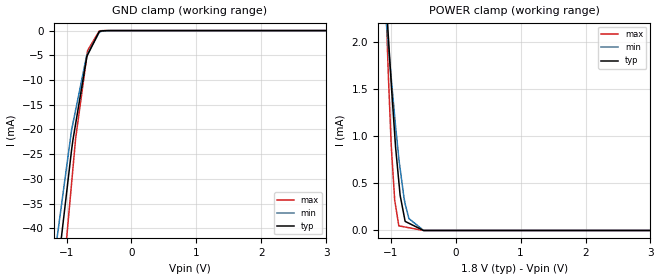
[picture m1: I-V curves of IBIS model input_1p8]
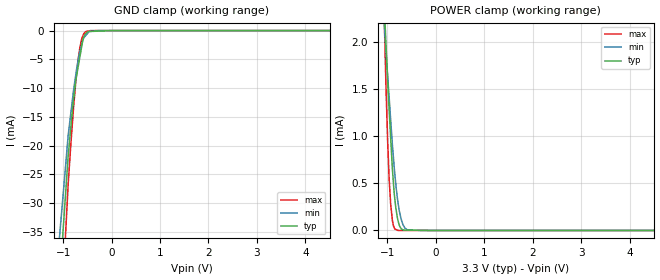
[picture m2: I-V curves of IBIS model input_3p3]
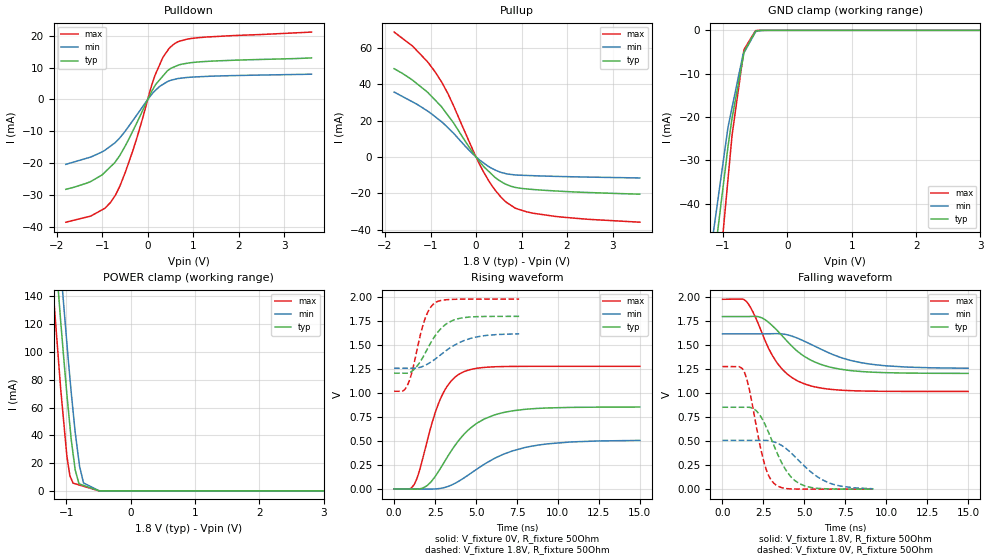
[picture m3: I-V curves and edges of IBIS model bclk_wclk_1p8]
|Texas Instruments Incorporated
| Low-Power Stereo DAC with 4 Outputs, HP/Speaker Amplifier and 3D Effects
| Marketing part#   Digital Voltage Range   Package-type   #pins
| TLV320DAC32IRHBR   1.1V - 3.6V   QFN   32
| TLV320DAC32IRHBRG4  1.1V - 3.6V   QFN   32
| TLV320DAC32IRHBT   1.1V - 3.6V   QFN   32
| TLV320DAC32IRHBTG4  1.1V - 3.6V   QFN   32
[IBIS Ver]   3.2
[File name]   tlv320dac32.ibs
|SIMDE Ver   V3.0 - 201101 - RHL4 - Build 457
[File Rev]   1.0
[Date]   9/15/2011
[Source]
| Texas Instruments Incorporated.
| Analog-eLab Design Center, HPA
| 12500 TI Blvd
| Dallas, TX -75243
| e-mail: elab_scm_ibis@list.ti.com
[Notes]   Revision History:
| Rev 1.0: 9/15/2011
| - Initial version of the model
| - Model generated from simulations in TISPICE
| - Model matched to SPICE simulation
| - C_comp although listed in numerical order of value are
|   obtained from varying PVT conditions. For PVT conditions for
|   each specific value refer the buffer description under
|   respective [Model]. IBIS model user is responsible for using
|   appropriate C_comp to simulate for Signal Integrity.
| - Model names with a trailing _1p8 contains the model for
|   1.8V [1.62V and 1.98V].Model names with a trailing _3p3
|   contains the model for 3.3V [3.0V and 3.6V].
[Disclaimer]
| This model is designed as an aid for customers of Texas Instruments.
| TI and its licensors and suppliers make no warranties, either expressed
| or implied, with respect to this  model, including the warranties of
| merchantability or fitness for a particular purpose. The model is
| provided solely on an "as is" basis. The entire risk as to its quality
| and performance is with the customer.
[Copyright]
 (C) Copyright 2011 Texas Instruments Incorporated.All rights reserved.
|   TLV320DAC32RHB
[Component]   TLV320DAC32RHB
[Manufacturer]   TI
[Package]   |32 QFN  -  RHB package
|   typ   min   max
R_pkg   0.09398   0.03334   0.13311
L_pkg   1.47574nH   0.53442nH   2.12719nH
C_pkg   0.15630pF   0.08976pF   0.19319pF
[Pin]  signal_name   model_name   R_pin   L_pin   C_pin
1   MCLK   INPUT   0.12336   1.96644nH  0.15900pF
2   BCLK   BCLK_WCLK   0.10740   1.68468nH  0.14850pF
3   WCLK   BCLK_WCLK   0.10191   1.58900nH  0.14672pF
4   DIN   INPUT   0.10100   1.57299nH  0.14533pF
5   LDO_SELECT   INPUT   0.10460   1.63539nH  0.15162pF
6   IOVSS   GND   0.11459   1.80939nH  0.15817pF
7   IOVDD   POWER   0.10859   1.70548nH  0.15212pF
8   SCL   SCL   0.12335   1.96583nH  0.16003pF
9   SDA   SDA   0.11930   1.89434nH  0.14528pF
10   LINEL   TERM   0.00029   0.05488nH  0.04405pF
11   LINEL   TERM   0.05460   0.78769nH  0.08976pF
12   LINEL   TERM   0.03334   0.53442nH  0.16822pF
13   LINER   TERM   0.03421   0.55249nH  0.17502pF
14   LINER   TERM   0.00029   0.05440nH  0.04408pF
15   MICBIAS   TERM   0.03710   0.57816nH  0.18724pF
16   MICBIAS   TERM   0.00029   0.05754nH  0.03663pF
17   DRVSS   GND   0.13014   2.07654nH  0.15925pF
18   DRVDD   POWER   0.05310   1.27721nH  0.19416pF
19   HPLOUT   TERM   0.10102   1.56409nH  0.15141pF
20   HPLCOM   TERM   0.10193   1.57999nH  0.15153pF
21   DRVSS   GND   0.05419   1.31855nH  0.20715pF
22   HPRCOM   TERM   0.11859   1.87140nH  0.17545pF
23   HPROUT   TERM   0.13311   2.12719nH  0.19319pF
24   DRVDD   POWER   0.07565   2.22477nH  0.22198pF
25   AVDD_DAC   POWER   0.12099   1.91764nH  0.14964pF
26   AVSS_DAC   GND   0.03485   0.58219nH  0.16642pF
27   AVSS_DAC   GND   0.00029   0.05439nH  0.04408pF
28   AVSS_DAC   GND   0.05222   0.75975nH  0.08772pF
29   AVSS_DAC   GND   0.05222   0.75975nH  0.08756pF
30   AVSS_DAC   GND   0.05686   0.82975nH  0.09264pF
31   _RESET   INPUT   0.10879   1.70768nH  0.15255pF
32   DVDD   POWER   0.06209   1.75808nH  0.19293pF
33   THERMAL_PAD   NC   0.00003   0.01397nH  0.12486pF
[Pin Mapping]  pulldown_ref pullup_ref gnd_clamp_ref power_clamp_ref
1   GNDBUS1   PWRBUS1
2   GNDBUS1   PWRBUS1
3   GNDBUS1   PWRBUS1
4   GNDBUS1   PWRBUS1
5   GNDBUS1   PWRBUS1
6   GNDBUS1   NC
7   NC   PWRBUS1
8   GNDBUS1   PWRBUS1
9   GNDBUS1   PWRBUS1
10   GNDBUS2   PWRBUS2
11   GNDBUS2   PWRBUS2
12   GNDBUS2   PWRBUS2
13   GNDBUS2   PWRBUS2
14   GNDBUS2   PWRBUS2
15   GNDBUS2   PWRBUS2
16   GNDBUS2   PWRBUS2
17   GNDBUS2   NC
18   NC   PWRBUS2
19   GNDBUS2   PWRBUS2
20   GNDBUS2   PWRBUS2
21   GNDBUS2   NC
22   GNDBUS2   PWRBUS2
23   GNDBUS2   PWRBUS2
24   NC   PWRBUS2
25   NC   PWRBUS3
26   GNDBUS3   NC
27   GNDBUS3   NC
28   GNDBUS3   NC
29   GNDBUS3   NC
30   GNDBUS3   NC
31   GNDBUS1   PWRBUS1
32   NC   PWRBUS4
33   NC   NC
|   Model Selectors
[Model Selector] INPUT
input_1p8   1.8V digital input
input_3p3   3.3V digital input
[Model Selector] BCLK_WCLK
bclk_wclk_1p8   1.8V digital I/O
bclk_wclk_3p3   3.3V digital I/O
[Model Selector] SCL
scl_1p8   1.8V digital input
scl_3p3   3.3V digital input
[Model Selector] SDA
sda_1p8  1.8V digital I/O_open_drain
sda_3p3  3.3V digital I/O_open_drain
[Model Selector] TERM
term_1-8V  1.8V nominal termination
term_3-3V  3.3V nominal termination
[Model] term_1-8V
Model_type Terminator
C_comp   1.0e-20F  1.0e-20F  1.0e-20F
|   typ   min   max
[Voltage Range]   1.8V   1.62V   1.98V
[POWER Clamp Reference]   1.8V   1.62V   1.98V
[GND Clamp Reference]   0V   0V   0V
|Ambient Temperature   25   85   -40
|Junction Temperature
[Temperature Range]   45   105   -40
[Model] term_3-3V
Model_type Terminator
C_comp   1.0e-20F  1.0e-20F  1.0e-20F
|   typ   min   max
[Voltage Range]   3.3V   3.0V   3.6V
[POWER Clamp Reference]   3.3V   3.0V   3.6V
[GND Clamp Reference]   0V   0V   0V
|Ambient Temperature   25   85   -40
|Junction Temperature
[Temperature Range]   45   105   -40
| Models and submodels in the file (10): input_1p8 (Input), input_3p3 (Input), bclk_wclk_1p8 (I/O), bclk_wclk_3p3 (I/O), scl_1p8 (Input), scl_3p3 (Input), sda_1p8 (I/O_open_drain), sda_3p3 (I/O_open_drain), term_1-8V (Terminator), term_3-3V (Terminator)
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|   input_1p8 Model
[Model]   input_1p8
Model_type   Input
Vinl = 0.54
Vinh = 1.26
|   typ   min   max
|   (nom PVT)   (fast PVT)   (slow PVT)
|C_comp from frequency sweep method (F=50MHz)
|Average
|C_comp   1.487e-12   1.450e-12   1.504e-12
|C_comp from LC tank measurement(L=1nH)
|Average
|Resonant Frequency(Hz)   4.930e+09   4.940e+09   4.930e+09
C_comp   1.043e-12   1.039e-12   1.043e-12
[Model spec]
|subparameter   typ   min   max
Vinl   0.54   0.486   0.594
Vinh   1.26   1.134   1.386
| Where nom  PVT is Nominal Process, 1.8V, 45C
|   Fast PVT is Strong Process,  1.98V, -40C
|   Slow PVT is Weak Process,   1.62V, 105C
[Voltage Range]   1.8   1.62   1.98
|Ambient Temperature   25   85   -40
|Junction Temperature
[Temperature Range]   45   105   -40
[Power Clamp Reference]   1.8   1.62   1.98
[GND Clamp Reference]   0   0   0
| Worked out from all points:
|   GND clamp passes 1 mA (typ) near -0.53 V on its own axis
|   POWER clamp passes 1 mA (typ) near -0.94 V on its own axis
[GND Clamp]
|   Voltage   I(typ)   I(min)   I(max)
-1.8V     -206.9mA   -110.5mA   -320.4mA
-1.152V   -50.18mA   -42.62mA   -64.48mA
-923.4mV  -24.31mA   -20.25mA   -31.11mA
-901.8mV  -22.19mA   -18.82mA   -27.97mA
-859.3mV  -18.84mA   -16.06mA   -21.82mA
-690.1mV  -5.53mA    -5.064mA   -5.476mA
-685.8mV  -5.19mA    -4.959mA   -5.059mA
-675.2mV  -4.913mA   -4.7mA     -4.033mA
-495mV    -199uA     -315.9uA   -54.51uA
-426.1mV  -36.83uA   -68.97uA   -5.36uA
-307.8mV  -1.051uA   -3.83uA    -71.36nA
3.6V      0A         0A         0A
[POWER Clamp]
|   Voltage   I(typ)   I(min)   I(max)
-1.8V     11.87mA    8.619mA    19.35mA
-1.085V   2.649mA    2.361mA    2.616mA
-1.039V   2.086mA    1.979mA    1.704mA
-990mV    1.542mA    1.604mA    881.4uA
-938.5mV  1.023mA    1.21mA     323.2uA
-923.4mV  874.4uA    1.094mA    257.8uA
-875.2mV  522uA      770.1uA    49.36uA
-855mV    374.8uA    656.9uA    46.74uA
-777.6mV  96.52uA    281.9uA    36.69uA
-719.3mV  76.6uA     126.4uA    29.12uA
-494.1mV  11.66nA    505.2nA    0A
3.6V      0A         0A         0A
|   input_3p3 Model
[Model]   input_3p3
Model_type   Input
Vinl = 0.99
Vinh = 2.31
|   typ   min   max
|   (nom PVT)   (fast PVT)   (slow PVT)
|C_comp from frequency sweep method (F=50MHz)
|Average
|C_comp   1.401e-12   1.371e-12   1.413e-12
|C_comp from LC tank measurement(L=1nH)
|Average
|Resonant Frequency(Hz)   5.100e+09   5.110e+09   5.090e+09
C_comp   9.748e-13   9.710e-13   9.787e-13
[model spec]
|subparameter   typ   min   max
Vinl   0.99   0.90   1.08
Vinh   2.31   2.10   2.52
| Where nom  PVT is Nominal Process, 3.3V, 45C
|   Fast PVT is Strong Process,  3.6V, -40C
|   Slow PVT is Weak Process,   3V, 105C
[Voltage Range]   3.3   3   3.6
|Ambient Temperature   25   85   -40
|Junction Temperature
[Temperature Range]   45   105   -40
[Power Clamp Reference]   3.3   3   3.6
[GND Clamp Reference]   0   0   0
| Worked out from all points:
|   GND clamp passes 1 mA (typ) near -0.57 V on its own axis
|   POWER clamp passes 1 mA (typ) near -0.93 V on its own axis
[GND Clamp]
|   Voltage   I(typ)   I(min)   I(max)
-3.3V     -1.459A    -1.317A    -1.646A
-1.49V    -95.13mA   -76.77mA   -122mA
-897.6mV  -21.78mA   -18.26mA   -26.74mA
-792mV    -12.42mA   -10.77mA   -14.02mA
-745.8mV  -8.948mA   -8.013mA   -9.431mA
-702mV    -6.825mA   -5.63mA    -5.815mA
-622.8mV  -2.986mA   -2.616mA   -1.616mA
-590.7mV  -1.43mA    -1.587mA   -839.1uA
-532.8mV  -508.5uA   -839.9uA   -172.5uA
-465mV    -161.8uA   -161.4uA   -53.2uA
-285mV    -98.74uA   -2.083uA   -3.877uA
6.6V      0A         0A         0A
[POWER Clamp]
|   Voltage   I(typ)   I(min)   I(max)
-3.3V     32.08mA    22.4mA     56.05mA
-1.089V   2.679mA    2.39mA     2.744mA
-1.03V    1.983mA    1.906mA    1.532mA
-993.6mV  1.586mA    1.634mA    934uA
-964.8mV  1.288mA    1.419mA    561.5uA
-932.4mV  983.8uA    1.176mA    280.4uA
-896.4mV  648.9uA    907.5uA    104uA
-864.6mV  429.3uA    705.3uA    36.05uA
-792mV    130.4uA    335uA      1.308uA
-681mV    8.006uA    64.67uA    29.85nA
-585mV    3.401uA    6.441uA    18.01nA
6.6V      0A         0A         0A
|   bclk_wclk_1p8 Model
[Model]   bclk_wclk_1p8
Model_type   I/O
Polarity   Non-Inverting
Enable   Active-Low
Vinl = 0.54
Vinh = 1.26
Vmeas = 0.9
Vref = 0.9
Cref = 10pF
Rref = 50
|   typ   min   max
|   (nom PVT)   (fast PVT)   (slow PVT)
|C_comp from frequency sweep method (F=14MHz)
|Average
|C_comp   3.261e-12   3.029e-12   3.353e-12
|ON state : BUFFER OUTPUT TURNED HIGH
|C_comp   4.573e-12   4.126e-12   4.742e-12
|OFF state: BUFFER IN HIGH IMPEDANCE
|C_comp   1.949e-12   1.931e-12   1.963e-12
|C_comp from LC tank measurement(L=1nH)
|Average
|Resonant Frequency(Hz)   4.330e+09   4.360e+09   4.290e+09
|C_comp   1.354e-12   1.336e-12   1.381e-12
|ON state : BUFFER OUTPUT TURNED HIGH
|Resonant Frequency(Hz)   4.230e+09   4.270e+09   4.160e+09
|C_comp   1.417e-12   1.391e-12   1.465e-12
|OFF state: BUFFER IN HIGH IMPEDANCE
|Resonant Frequency(Hz)   4.430e+09   4.450e+09   4.420e+09
C_comp   1.292e-12   1.280e-12   1.298e-12
[Model spec]
|subparameter   typ   min   max
Vinl   0.54   0.486   0.594
Vinh   1.26   1.134   1.386
| Where nom  PVT is Nominal Process, 1.8V, 45C
|   Fast PVT is Strong Process,  1.98V, -40C
|   Slow PVT is Weak Process,   1.62V, 105C
[Voltage Range]   1.8   1.62   1.98
|Ambient Temperature   25   85   -40
|Junction Temperature
[Temperature Range]   45   105   -40
[Pullup Reference]   1.8   1.62   1.98
[Pulldown Reference]   0   0   0
[Power Clamp Reference]   1.8   1.62   1.98
[GND Clamp Reference]   0   0   0
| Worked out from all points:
|   slope of the pulldown table from 0 to 0.27 V, typ, clamps not added: 42.9 ohm
|   slope of the pullup table from 0 to 0.27 V, typ, clamps not added: 35 ohm
|   GND clamp passes 1 mA (typ) near -0.52 V on its own axis
|   POWER clamp passes 1 mA (typ) near -0.55 V on its own axis
|   falling waveform, V_fixture 1.8V, R_fixture 50Ohm: 20-80 % time 2.45ns typ, 3.16ns min, 1.86ns max; typ from 1.8 V to 1.21 V
|   rising waveform, V_fixture 0V, R_fixture 50Ohm: 20-80 % time 2.38ns typ, 3.26ns min, 1.42ns max; typ from 0 V to 0.854 V
|   rising waveform, V_fixture 1.8V, R_fixture 50Ohm: 20-80 % time 1.32ns typ, 1.94ns min, 839ps max; typ from 1.21 V to 1.8 V
|   falling waveform, V_fixture 0V, R_fixture 50Ohm: 20-80 % time 1.41ns typ, 2.04ns min, 918ps max; typ from 0.854 V to 0 V
[Pulldown]
|   Voltage   I(typ)   I(min)   I(max)
-1.8V     -28.16mA   -20.33mA   -38.46mA
-1.247V   -25.67mA   -18.02mA   -36.51mA
-938.5mV  -22.76mA   -15.87mA   -34.05mA
-708.8mV  -19.47mA   -13.42mA   -29.97mA
-495mV    -14.59mA   -9.946mA   -22.93mA
-326.7mV  -9.861mA   -6.597mA   -16.03mA
160.4mV   4.355mA    2.755mA    7.566mA
348.5mV   7.585mA    4.859mA    13.5mA
601.9mV   10.33mA    6.349mA    17.62mA
855.4mV   11.33mA    6.885mA    18.88mA
1.277V    11.92mA    7.225mA    19.56mA
3.6V      13.02mA    7.925mA    21.12mA
[GND Clamp]
|   Voltage   I(typ)   I(min)   I(max)
-1.8V     -194.5mA   -121.1mA   -306.7mA
-1.146V   -54.38mA   -46.2mA    -70.27mA
-1.127V   -51.62mA   -44.11mA   -67.11mA
-923.4mV  -26.89mA   -22.39mA   -34.39mA
-867.6mV  -20.95mA   -18.36mA   -25.42mA
-859.3mV  -20.24mA   -17.76mA   -24.13mA
-690.1mV  -6.434mA   -5.598mA   -6.056mA
-675.2mV  -5.215mA   -5.196mA   -4.46mA
-671.4mV  -4.906mA   -5.094mA   -4.368mA
-495mV    -219.7uA   -348.7uA   -60.12uA
-307.8mV  -1.158uA   -4.217uA   -78.64nA
3.6V      0A         0A         0A
[Pullup]
|   Voltage   I(typ)   I(min)   I(max)
-1.8V     48.47mA    35.64mA    68.56mA
-1.4V     42.25mA    30.29mA    60.99mA
-1.069V   35.61mA    25.29mA    52.35mA
-895mV    31.14mA    22.03mA    46.57mA
-619.7mV  22.9mA     16.09mA    34.88mA
-72.9mV   2.538mA    1.705mA    3.995mA
164.3mV   -5.105mA   -3.246mA   -8.174mA
415.8mV   -11.19mA   -7.11mA    -18.09mA
669.2mV   -15.13mA   -9.24mA    -24.94mA
889mV     -16.83mA   -9.911mA   -28.39mA
1.277V    -17.9mA    -10.3mA    -30.98mA
3.6V      -20.43mA   -11.53mA   -35.81mA
[POWER Clamp]
|   Voltage   I(typ)   I(min)   I(max)
-1.8V     565.3mA    591.8mA    531.1mA
-1.217V   197.8mA    236.3mA    150.6mA
-1.129V   146.1mA    182.9mA    97.8mA
-1.044V   97.09mA    135.2mA    50.98mA
-990mV    68.2mA     105mA      24.23mA
-946.4mV  47.32mA    81.95mA    11.12mA
-896.9mV  27.05mA    57.81mA    5.6mA
-864mV    15.33mA    42.54mA    5.145mA
-804.6mV  5.118mA    21.06mA    4.326mA
-733.9mV  3.982mA    5.74mA     3.35mA
-494.1mV  142.4uA    165.8uA    53.11uA
3.6V      0A         0A         0A
[Ramp]
R_load = 50
|   typ   min   max
dV/dt_r   0.512338/2.37418e-09   0.30364/3.239e-09   0.767305/1.41475e-09
dV/dt_f   0.355561/2.44835e-09   0.215507/3.14651e-09   0.576698/1.85932e-09
[Falling Waveform]
V_fixture = 1.8V
V_fixture_min = 1.62V
V_fixture_max = 1.98V
R_fixture = 50Ohm
|   Time   V(typ)   V(min)   V(max)
0s        1.8V       1.62V      1.98V
1.452ns   1.8V       1.62V      1.959V
1.86ns    1.802V     1.62V      1.848V
2.416ns   1.785V     1.62V      1.628V
3.296ns   1.662V     1.621V     1.327V
4.052ns   1.524V     1.606V     1.187V
4.976ns   1.387V     1.545V     1.1V
6.464ns   1.277V     1.424V     1.044V
8.492ns   1.227V     1.318V     1.024V
15ns      1.207V     1.261V     1.019V
[Rising Waveform]
V_fixture = 0V
V_fixture_min = 0V
V_fixture_max = 0V
R_fixture = 50Ohm
|   Time   V(typ)   V(min)   V(max)
0s        2.183nV    21.82nV    577pV
1.228ns   -2.315mV   -48.69uV   47.35mV
1.544ns   346.2uV    -766.4uV   189.8mV
2.024ns   36.64mV    -1.82mV    505.1mV
2.8ns     207.3mV    5.094mV    929.3mV
3.408ns   375.7mV    33.87mV    1.11V
4.148ns   547.8mV    101.7mV    1.214V
5.58ns    735.1mV    265.7mV    1.268V
8ns       830.4mV    432.3mV    1.278V
15ns      853.9mV    506.1mV    1.279V
[Rising Waveform]
V_fixture = 1.8V
V_fixture_min = 1.62V
V_fixture_max = 1.98V
R_fixture = 50Ohm
|   Time   V(typ)   V(min)   V(max)
0s        1.207V     1.259V     1.019V
540ps     1.207V     1.259V     1.022V
828ps     1.208V     1.259V     1.088V
1.1ns     1.23V      1.258V     1.226V
1.764ns   1.376V     1.279V     1.711V
2.436ns   1.581V     1.346V     1.934V
3.056ns   1.704V     1.427V     1.971V
3.884ns   1.774V     1.518V     1.978V
5.424ns   1.798V     1.596V     1.98V
7.632ns   1.8V       1.618V     1.98V
[Falling Waveform]
V_fixture = 0V
V_fixture_min = 0V
V_fixture_max = 0V
R_fixture = 50Ohm
|   Time   V(typ)   V(min)   V(max)
0s        854.2mV    508.4mV    1.279V
1.332ns   854.2mV    508.4mV    1.222V
1.636ns   853.6mV    508.4mV    1.042V
1.96ns    832.1mV    508.4mV    752.9mV
2.54ns    695.1mV    508.7mV    277.7mV
3.252ns   410.3mV    486.7mV    45.35mV
4.14ns    136.4mV    385.7mV    3.011mV
5.032ns   33.31mV    235.9mV    934uV
6.672ns   2.332mV    55.6mV     279.7uV
9.208ns   239.6uV    4.185mV    52.28uV
